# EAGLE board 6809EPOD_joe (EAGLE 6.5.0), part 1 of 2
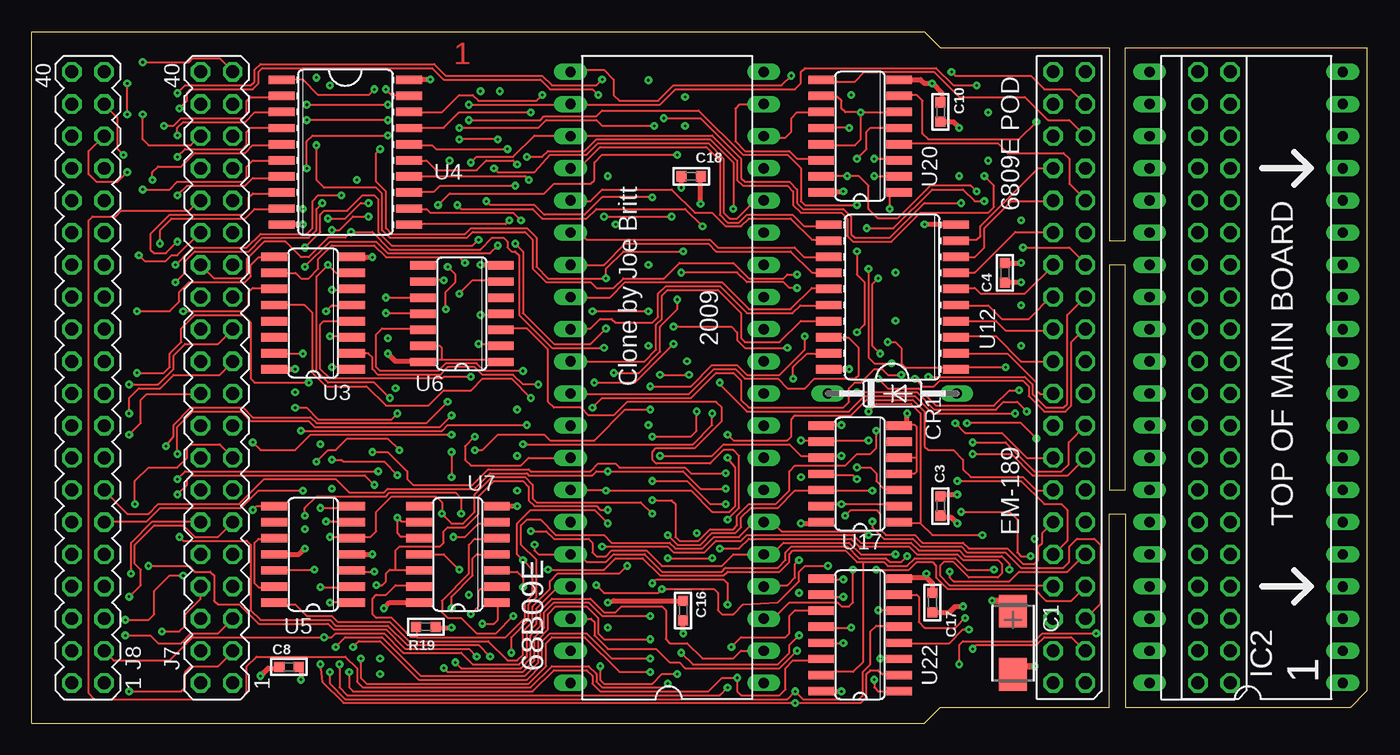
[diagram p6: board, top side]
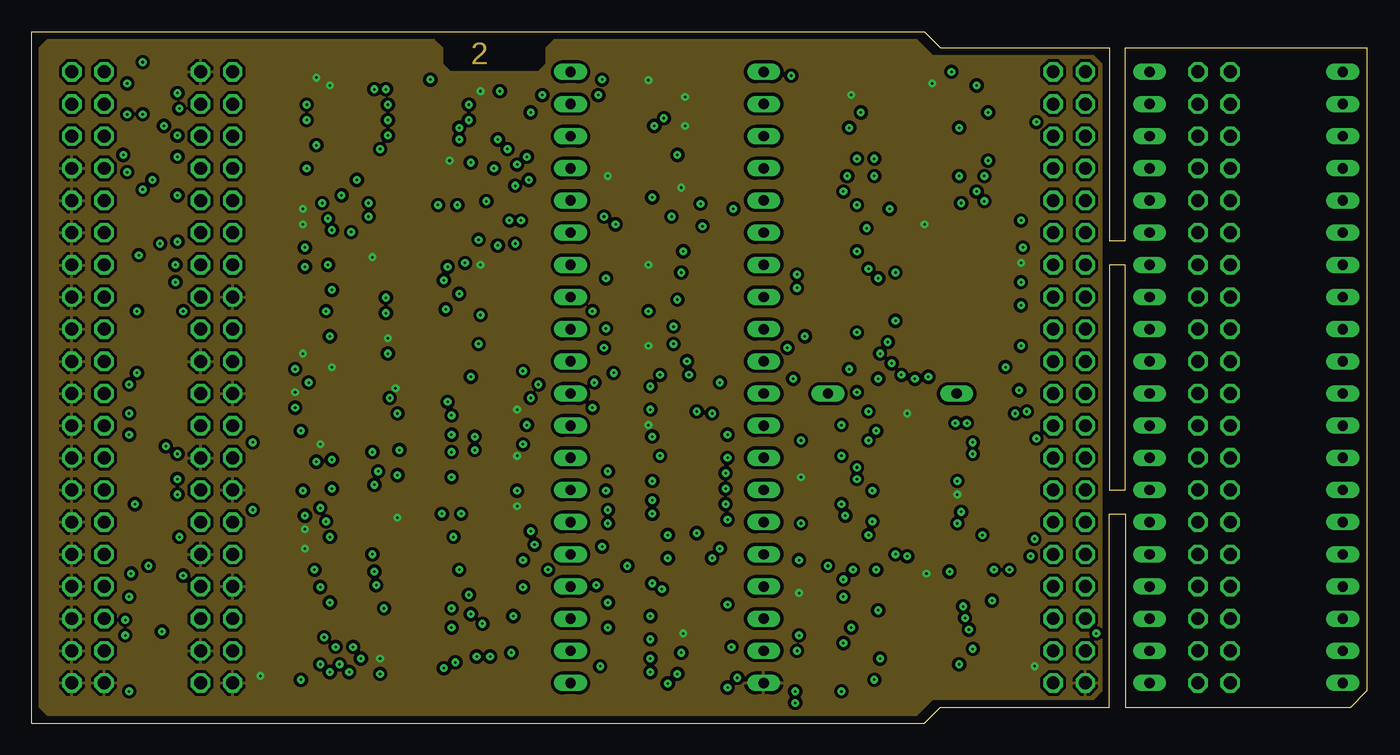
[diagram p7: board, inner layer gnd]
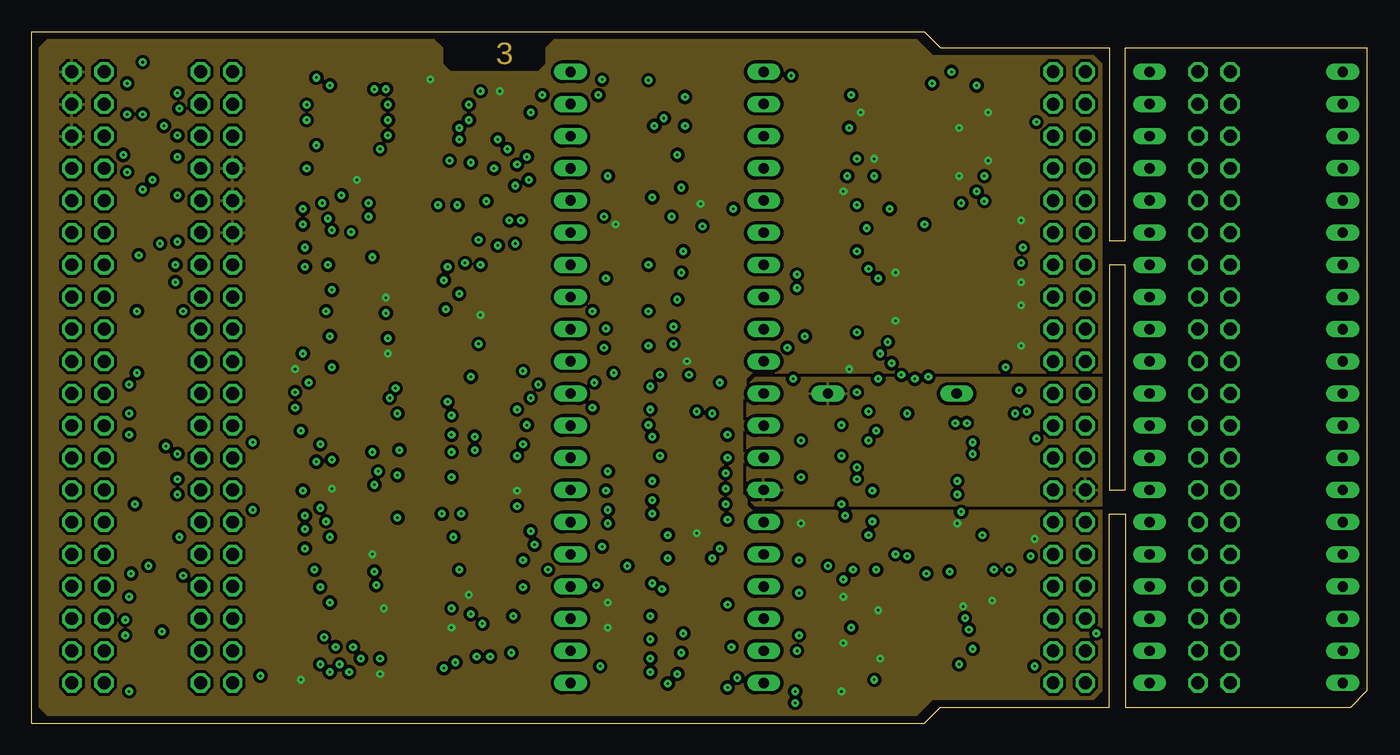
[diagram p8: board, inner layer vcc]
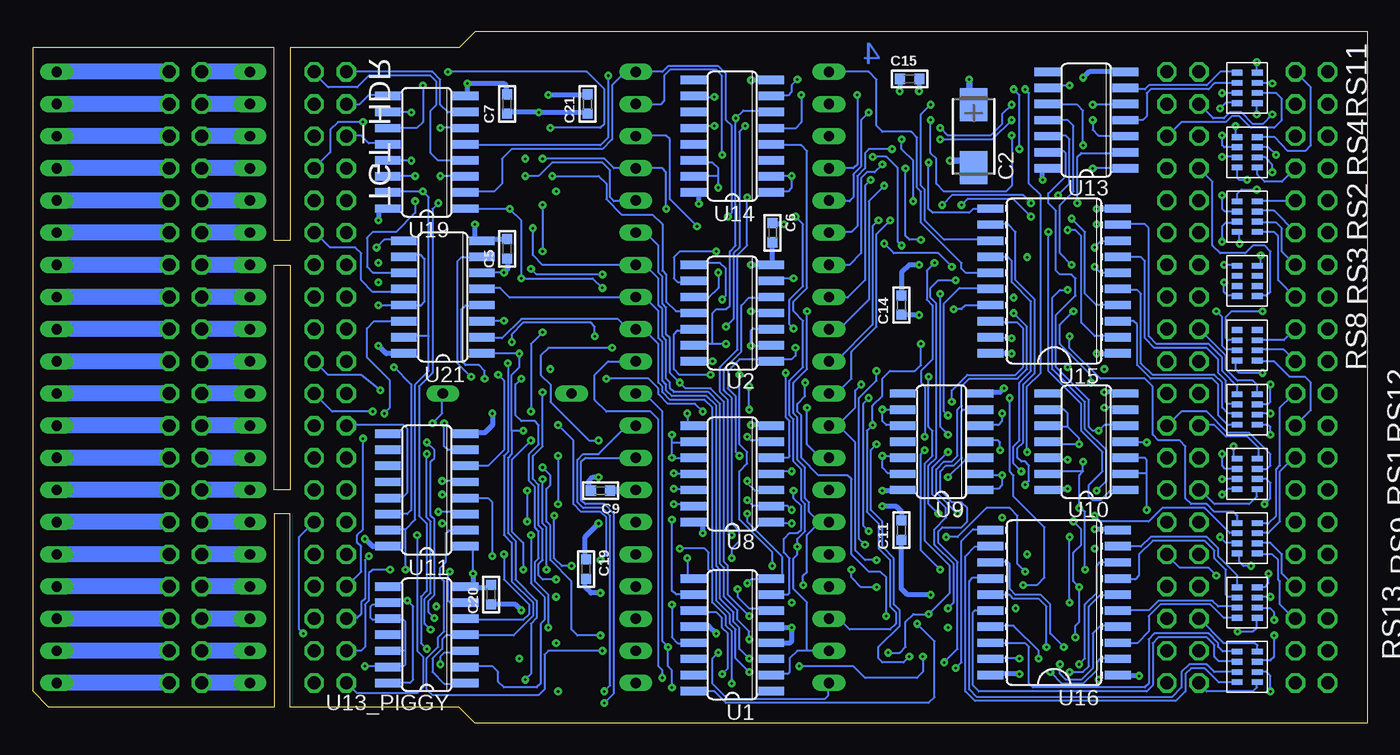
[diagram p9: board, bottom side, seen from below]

Size 105.41 x 54.61 mm. Coordinates in mm from the lower left corner, seen from the top.
Outline: 0,0 0,54.61 70.48,54.61 71.75,53.34 85.09,53.34 85.09,38.1 86.36,38.1 86.36,53.34 105.41,53.34 105.41,2.54 104.14,1.27 86.36,1.27 86.36,16.51 85.09,16.51 85.09,1.27 71.75,1.27 70.48,0 0,0
Outline: 85.09,18.41 86.36,18.41 86.36,36.2 85.09,36.2 85.09,18.41
Copper layers (1*4*5*16): Top 0.035mm / dielectric 1.5mm / gnd 0.035mm / dielectric 0.15mm / vcc 0.035mm / dielectric 0.2mm / Bottom 0.035mm
Design rules "default": minimum track width 6mil, minimum drill 8mil, track to track 6mil, track to pad 6mil, pad to pad 6mil, via to via 10mil, smd to smd 6mil, copper to edge 18mil, drill to drill 6mil, minimum pad ring 10mil, minimum via ring 8mil, stop-mask expansion 4mil, vias tented up to drill 8mil, thermal gap 10mil

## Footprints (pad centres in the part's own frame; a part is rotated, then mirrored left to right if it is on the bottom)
DIL40 = drill 0.813 long: 1 -24.13,-7.62; 2 -21.59,-7.62; 3 -19.05,-7.62; 4 -16.51,-7.62; 5 -13.97,-7.62; 6 -11.43,-7.62; 7 -8.89,-7.62; 8 -6.35,-7.62; 9 -3.81,-7.62; 10 -1.27,-7.62; 11 1.27,-7.62; 12 3.81,-7.62; 13 6.35,-7.62; 14 8.89,-7.62; 15 11.43,-7.62; 16 13.97,-7.62; 17 16.51,-7.62; 18 19.05,-7.62; 19 21.59,-7.62; 20 24.13,-7.62; 21 24.13,7.62; 22 21.59,7.62; 23 19.05,7.62; 24 16.51,7.62; 25 13.97,7.62; 26 11.43,7.62; 27 8.89,7.62; 28 6.35,7.62; 29 3.81,7.62; 30 1.27,7.62; 31 -1.27,7.62; 32 -3.81,7.62; 33 -6.35,7.62; 34 -8.89,7.62; 35 -11.43,7.62; 36 -13.97,7.62; 37 -16.51,7.62; 38 -19.05,7.62; 39 -21.59,7.62; 40 -24.13,7.62
CT6032 = smd 2.6 x 2.2: + 2.5,0; - -2.5,0
C0603 = smd 0.8 x 0.8: 1 -0.762,0; 2 0.762,0
DO35-10 = drill 0.813 long: A 5.08,0; C -5.08,0
HDR40 = drill 1.016 octagon: 1 -24.13,-1.27; 2 -21.59,-1.27; 3 -19.05,-1.27; 4 -16.51,-1.27; 5 -13.97,-1.27; 6 -11.43,-1.27; 7 -8.89,-1.27; 8 -6.35,-1.27; 9 -3.81,-1.27; 10 -1.27,-1.27; 11 1.27,-1.27; 12 3.81,-1.27; 13 6.35,-1.27; 14 8.89,-1.27; 15 11.43,-1.27; 16 13.97,-1.27; 17 16.51,-1.27; 18 19.05,-1.27; 19 21.59,-1.27; 20 24.13,-1.27; 21 24.13,1.27; 22 21.59,1.27; 23 19.05,1.27; 24 16.51,1.27; 25 13.97,1.27; 26 11.43,1.27; 27 8.89,1.27; 28 6.35,1.27; 29 3.81,1.27; 30 1.27,1.27; 31 -1.27,1.27; 32 -3.81,1.27; 33 -6.35,1.27; 34 -8.89,1.27; 35 -11.43,1.27; 36 -13.97,1.27; 37 -16.51,1.27; 38 -19.05,1.27; 39 -21.59,1.27; 40 -24.13,1.27
MA20-2 = drill 1.016 octagon: 1 -24.13,-1.27; 2 -24.13,1.27; 3 -21.59,-1.27; 4 -21.59,1.27; 5 -19.05,-1.27; 6 -19.05,1.27; 7 -16.51,-1.27; 8 -16.51,1.27; 9 -13.97,-1.27; 10 -13.97,1.27; 11 -11.43,-1.27; 12 -11.43,1.27; 13 -8.89,-1.27; 14 -8.89,1.27; 15 -6.35,-1.27; 16 -6.35,1.27; 17 -3.81,-1.27; 18 -3.81,1.27; 19 -1.27,-1.27; 20 -1.27,1.27; 21 1.27,-1.27; 22 1.27,1.27; 23 3.81,-1.27; 24 3.81,1.27; 25 6.35,-1.27; 26 6.35,1.27; 27 8.89,-1.27; 28 8.89,1.27; 29 11.43,-1.27; 30 11.43,1.27; 31 13.97,-1.27; 32 13.97,1.27; 33 16.51,-1.27; 34 16.51,1.27; 35 19.05,-1.27; 36 19.05,1.27; 37 21.59,-1.27; 38 21.59,1.27; 39 24.13,-1.27; 40 24.13,1.27
R0603 = smd 0.8 x 0.8: 1 -0.762,0; 2 0.762,0
V8V = smd 0.45 x 0.85: R1A -1.2,-0.8; R1B -1.2,0.8; R2A -0.4,-0.8; R2B -0.4,0.8; R3A 0.4,-0.8; R3B 0.4,0.8; R4A 1.2,-0.8; R4B 1.2,0.8
SO16 = smd 0.66 x 2.032: 1 -4.445,-3.073; 2 -3.175,-3.073; 3 -1.905,-3.073; 4 -0.635,-3.073; 5 0.635,-3.073; 6 1.905,-3.073; 7 3.175,-3.073; 8 4.445,-3.073; 9 4.445,3.073; 10 3.175,3.073; 11 1.905,3.073; 12 0.635,3.073; 13 -0.635,3.073; 14 -1.905,3.073; 15 -3.175,3.073; 16 -4.445,3.073
SO14 = smd 0.66 x 2.032: 1 -3.81,-3.073; 2 -2.54,-3.073; 3 -1.27,-3.073; 4 0,-3.073; 5 1.27,-3.073; 6 2.54,-3.073; 7 3.81,-3.073; 8 3.81,3.073; 9 2.54,3.073; 10 1.27,3.073; 11 0,3.073; 12 -1.27,3.073; 13 -2.54,3.073; 14 -3.81,3.073
SO20W = smd 0.66 x 2.032: 1 -5.715,-5.029; 2 -4.445,-5.029; 3 -3.175,-5.029; 4 -1.905,-5.029; 5 -0.635,-5.029; 6 0.635,-5.029; 7 1.905,-5.029; 8 3.175,-5.029; 9 4.445,-5.029; 10 5.715,-5.029; 11 5.715,5.029; 12 4.445,5.029; 13 3.175,5.029; 14 1.905,5.029; 15 0.635,5.029; 16 -0.635,5.029; 17 -1.905,5.029; 18 -3.175,5.029; 19 -4.445,5.029; 20 -5.715,5.029

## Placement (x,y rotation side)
68B09E  [DIL40]  50.16,27.3 90 top
C1  33uF  [CT6032]  77.47,6.35 90 top
C2  33uF  [CT6032]  31.12,46.35 90 bottom
C3  .1uF  [C0603]  71.75,17.14 90 top
C4  .1uF  [C0603]  76.83,35.56 90 top
C5  .1uF  [C0603]  67.94,37.46 90 bottom
C6  .1uF  [C0603]  46.99,38.73 270 bottom
C7  .1uF  [C0603]  67.94,48.89 90 bottom
C8  .1uF  [C0603]  20.32,4.44 180 top
C9  .1uF  [C0603]  60.58,18.36 180 bottom
C10  .1uF  [C0603]  71.75,48.26 90 top
C11  .1uF  [C0603]  36.83,15.24 90 bottom
C14  .1uF  [C0603]  36.83,33.02 90 bottom
C15  .1uF  [C0603]  36.17,50.88 0 bottom
C16  .1uF  [C0603]  51.44,8.89 270 top
C17  .1uF  [C0603]  71.12,9.53 90 top
C18  .1uF  [C0603]  52.07,43.18 180 top
C19  .1uF  [C0603]  61.72,12.17 270 bottom
C20  .1uF  [C0603]  69.22,10.16 90 bottom
C21  .1uF  [C0603]  61.59,48.89 90 bottom
CR1  1N4148  [DO35-10]  67.94,26.04 0 top
IC1  [DIL40]  95.89,27.3 90 top
IC2  [HDR40]  93.34,27.3 90 top
J7  [MA20-2]  14.61,27.3 90 top
J8  [MA20-2]  4.44,27.3 90 top
R19  10k  [R0603]  31.12,7.62 0 top
RS1  75  [V8V]  9.53,14.61 90 bottom
RS2  22  [V8V]  9.53,40 90 bottom
RS3  75  [V8V]  9.53,29.84 90 bottom
RS4  22  [V8V]  9.53,45.09 90 bottom
RS8  75  [V8V]  9.53,34.92 90 bottom
RS9  75  [V8V]  9.53,19.68 270 bottom
RS10  75  [V8V]  9.53,4.44 270 bottom
RS11  75  [V8V]  9.53,50.16 270 bottom
RS12  75  [V8V]  9.53,24.77 270 bottom
RS13  75  [V8V]  9.53,9.53 270 bottom
TGT_HDR  [HDR40]  81.91,27.3 90 top
U1  74LS75D  [SO16]  50.16,6.99 90 bottom
U2  74LS27D  [SO14]  50.16,32.38 90 bottom
U3  74LS367D  [SO16]  22.22,32.38 90 top
U4  74LS245DW  [SO20W]  24.77,45.09 270 top
U5  74LS73D  [SO14]  22.22,13.34 90 top
U6  74LS74D  [SO14]  33.96,32.33 90 top
U7  74LS32D  [SO14]  33.66,13.34 90 top
U8  74LS00D  [SO14]  50.16,19.68 90 bottom
U9  74LS00D  [SO14]  33.66,22.22 90 bottom
U10  74LS10D  [SO14]  22.22,22.22 90 bottom
U11  74LS367D  [SO16]  74.3,18.41 90 bottom
U12  74LS245DW  [SO20W]  67.94,33.66 90 top
U13  74LS04D  [SO14]  22.22,47.62 90 bottom
U13_PIGGY  74LS08D  [SO14]  74.3,6.99 90 bottom
U14  74LS367D  [SO16]  50.16,46.35 90 bottom
U15  74LS244DW  [SO20W]  24.77,34.92 90 bottom
U16  74LS244DW  [SO20W]  24.77,9.53 90 bottom
U17  74LS32D  [SO14]  65.41,19.68 90 top
U19  74LS257D  [SO16]  74.3,45.09 90 bottom
U20  74LS257D  [SO16]  65.41,46.35 90 top
U21  74LS257D  [SO16]  73.03,33.66 90 bottom
U22  74LS257D  [SO16]  65.41,6.99 90 top

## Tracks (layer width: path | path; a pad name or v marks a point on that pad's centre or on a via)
A0  (via drill 0.2)
  Top 0.152: v22.78,4.65 22.94,3.28 24.61,1.6 v60.27,1.6 65.46,1.6 65.91,2.06 65.91,3.89 66.22,4.19 66.83,4.19 67.13,3.89 68.4,3.89 U22.2
  Bottom 0.152: U16.8 19.76,12.73 21.11,12.73 21.41,12.42 21.41,10.29 22.33,9.37 22.33,5.1 v22.78,4.65 | v60.27,1.6 59.51,2.36 59.51,16.54 60.27,17.3 61.8,17.3 62.1,17.6 62.1,20.65 61.8,20.95 68B09E.8
A1  (via drill 0.2)
  Top 0.152: v23.55,4.04 23.55,3.12 24.77,1.91 59.66,1.91 v60.27,2.51 60.88,1.91 65.3,1.91 65.61,2.21 65.61,4.04 66.22,4.65 66.22,7.24 66.67,7.7 68.5,7.7 68.5,7.65 U22.5
  Bottom 0.152: U16.6 19.76,10.13 21.11,10.13 22.02,9.22 22.02,4.5 22.48,4.04 v23.55,4.04 | v60.27,2.51 59.82,2.97 59.82,16.38 60.43,16.99 61.95,16.99 62.41,17.45 62.41,20.8 61.95,21.26 60.73,21.26 58.45,23.55 57.84,23.55 68B09E.9
A2  (via drill 0.2)
  Top 0.152: v24.31,4.65 24.31,2.82 24.92,2.21 54.33,2.21 v54.94,2.82 | v55.24,6.02 56.01,6.78 59.51,6.78 59.82,7.09 59.82,8.46 60.27,8.92 62.25,8.92 62.28,8.89 U22.11
  Bottom 0.152: U16.4 19.81,7.7 21.11,7.7 21.72,7.09 21.72,4.34 22.63,3.43 23.85,3.43 24.31,3.89 v24.31,4.65 | v54.94,2.82 54.94,4.19 55.24,4.5 v55.24,6.02 55.7,6.48 55.7,24.61 57.07,25.98 57.68,25.98 68B09E.10
A3  (via drill 0.2)
  Top 0.152: v25.07,4.04 25.07,2.82 25.38,2.51 39.55,2.51 41.22,4.19 43.81,4.19 44.27,3.73 44.27,3.12 44.88,2.51 53.42,2.51 54.48,3.58 v55.7,3.58 55.7,2.51 56.01,2.21 59.05,2.21 59.51,2.67 59.51,4.34 60.12,4.95 62.15,4.95 U22.14
  Bottom 0.152: U16.2 19.76,5.1 21.11,5.1 21.41,4.8 21.41,4.19 22.48,3.12 24.15,3.12 v25.07,4.04 | v55.7,3.58 55.7,4.19 56.01,4.5 56.01,24 56.62,24.61 60.12,24.61 61.04,25.53 61.04,27.51 59.97,28.57 68B09E.11
A4  (via drill 0.2)
  Top 0.152: v48.84,4.04 46.41,4.04 43.66,6.78 41.07,6.78 40.62,6.33 40.62,4.5 39.24,3.12 26.44,3.12 25.98,3.58 v25.98,5.1
  Bottom 0.152: U16.17 29.87,7.7 27.96,7.7 25.98,5.71 v25.98,5.1 | U21.2 69.88,30.4 68.35,30.4 66.83,31.93 59.21,31.93 58.45,31.17 57.84,31.17 68B09E.12 57.73,31.12 57.68,31.17 57.07,31.01 56.01,29.95 56.01,26.9 55.7,26.59 55.7,26.14 55.09,25.53 52.35,25.53 51.74,24.92 51.74,12.27 51.44,11.96 51.44,9.68 50.37,8.61 50.37,7.85 49.91,7.39 49.91,5.1 v48.84,4.04
A5  (via drill 0.2)
  Top 0.152: v48.84,5.1 45.8,5.1 43.81,7.09 40.92,7.09 40.31,6.48 40.31,4.65 39.09,3.43 30.56,3.43 27.51,6.48 25.83,6.48 v25.38,6.02
  Bottom 0.152: U16.15 29.82,10.13 28.27,10.13 27.96,9.83 25.98,9.83 25.38,9.22 v25.38,6.02 | U21.5 69.88,34.37 68.5,34.37 67.74,33.6 57.89,33.6 68B09E.13 57.73,33.66 57.68,33.6 57.07,33.6 56.01,32.54 56.01,30.4 55.7,30.1 55.7,27.05 55.4,26.75 55.4,26.29 54.94,25.83 52.2,25.83 51.44,25.07 51.44,12.42 51.13,12.12 51.13,9.83 50.06,8.76 50.06,8 49.61,7.54 49.61,5.87 v48.84,5.1
A6  (via drill 0.2)
  Top 0.152: v75.21,41.22 74.45,41.22 73.53,42.14 71.09,42.14 68.05,39.09 v65.91,39.09 | v48.84,6.63 45.19,6.63 44.73,7.09 44.73,8.31 43.81,9.22 41.38,9.22 40.77,8.61 40.77,7.39 40,6.63 40,4.8 38.94,3.73 30.71,3.73 27.66,6.78 24.77,6.78 v24,6.02
  Bottom 0.152: U16.13 29.82,12.73 28.42,12.73 28.27,12.57 28.27,10.59 27.81,10.13 25.83,10.13 25.07,9.37 25.07,7.09 v24,6.02 | U21.11 76.12,35.59 78.56,35.59 79.02,36.04 79.02,38.33 78.56,38.79 76.73,38.79 75.21,40.31 v75.21,41.22 | v65.91,39.09 65.91,36.96 65.15,36.2 68B09E.14 57.07,36.2 56.01,35.13 56.01,32.99 55.7,32.69 55.7,30.56 55.4,30.25 55.4,27.2 55.09,26.9 55.09,26.44 54.79,26.14 52.05,26.14 51.13,25.22 51.13,12.57 50.82,12.27 50.82,9.98 49.76,8.92 49.76,8.15 48.84,7.24 v48.84,6.63
A7  (via drill 0.2)
  Top 0.152: v77.65,24.46 71.09,24.46 69.72,25.83 65.76,25.83 64.54,24.61 56.46,24.61 54.33,26.75 v54.33,26.9 | v48.84,8.46 45.03,8.46 43.97,9.53 41.22,9.53 40.46,8.76 40.46,7.54 39.7,6.78 39.7,4.95 38.79,4.04 32.84,4.04 v32.54,4.34
  Bottom 0.152: U16.11 29.87,15.32 31.17,15.32 32.08,14.4 32.08,4.8 v32.54,4.34 | 68B09E.15 57.84,38.79 57.07,38.79 56.01,37.72 56.01,35.59 55.7,35.28 55.7,33.15 55.4,32.84 55.4,30.71 55.09,30.4 55.09,27.66 v54.33,26.9 53.87,26.44 51.89,26.44 50.82,25.38 50.82,12.73 50.52,12.42 50.52,10.13 v48.84,8.46 | U21.14 78.44,31.75 79.02,31.17 79.02,28.88 77.19,27.05 77.19,24.92 v77.65,24.46
A8  (via drill 0.2)
  Top 0.152: U20.2 68.45,43.2 v66.52,43.2 | v21.56,37.57 22.78,38.79 22.78,40.16 23.09,40.46 24.92,40.46 26.14,41.68 27.05,41.68 27.36,41.38 27.36,38.79 28.42,37.72 34.82,37.72 v35.28,38.18 | v36.5,43.81 36.8,43.51 39.7,43.51 40.92,44.88 43.81,44.88 44.73,45.8 53.42,45.8 54.63,44.58 54.63,40.31 55.09,39.85 55.7,39.85 57.07,41.22 57.68,41.22 57.73,41.27 68B09E.16
  Bottom 0.152: 68B09E.16 57.84,41.22 59.51,41.22 59.82,41.53 59.82,43.66 60.43,44.27 64.39,44.27 65.46,43.2 v66.52,43.2 | U15.8 19.81,38.02 21.11,38.02 v21.56,37.57 | v35.28,38.18 36.2,38.18 36.5,38.48 v36.5,43.81
A9  (via drill 0.2)
  Top 0.152: U20.5 68.45,47.02 66.22,47.02 65.91,46.71 65.91,45.34 v65.15,44.58 | v21.56,36.04 23.55,38.02 27.2,38.02 28.12,37.11 36.2,37.11 v36.8,37.72 | v39.09,44.73 40.31,44.73 40.77,45.19 43.66,45.19 44.58,46.1 53.57,46.1 55.4,44.27 v55.4,40.62
  Bottom 0.152: v65.15,44.58 60.27,44.58 59.51,43.81 68B09E.17 55.7,43.81 55.4,43.51 v55.4,40.62 | U15.6 21.08,35.56 v21.56,36.04 | v36.8,37.72 37.11,38.02 37.11,43.81 38.02,44.73 v39.09,44.73
A10  (via drill 0.2)
  Top 0.152: 68B09E.18 57.89,46.25 59.51,46.25 59.97,46.71 59.97,47.78 60.43,48.23 62.31,48.23 U20.11 | v23.39,39.85 24.77,39.85 25.98,41.07 v26.59,41.07 | v33.6,40.92 33.91,40.62 39.55,40.62 40.31,39.85 43.81,39.85 44.58,40.62 51.59,40.62 v52.96,39.24
  Bottom 0.152: U15.4 21.44,33.02 22.33,33.91 22.33,38.79 v23.39,39.85 | v26.59,41.07 27.2,41.68 32.84,41.68 v33.6,40.92 | v52.96,39.24 55.09,41.38 55.09,46.1 55.4,46.41 57.68,46.41 57.73,46.35 68B09E.18
A11  (via drill 0.2)
  Top 0.152: U20.14 62.2,44.58 60.43,44.58 59.82,45.19 56.31,45.19 55.55,45.95 55.55,48.54 55.85,48.84 57.73,48.84 68B09E.19 | v23.7,38.94 24.31,38.94 25.38,40 v26.59,40 | v32.08,40.92 32.99,41.83 40.46,41.83 41.22,42.6 44.12,42.6 44.42,42.9 44.42,44.27 45.03,44.88 v50.98,44.88
  Bottom 0.152: U15.2 20.27,30.48 20.5,30.56 21.56,30.56 22.63,31.62 22.63,38.48 23.09,38.94 v23.7,38.94 | v26.59,40 27.96,41.38 31.62,41.38 v32.08,40.92 | v50.98,44.88 50.98,51.13 51.44,51.59 55.09,51.59 55.55,51.13 55.55,49.15 55.85,48.84 57.84,48.84 68B09E.19
A12  (via drill 0.2)
  Top 0.152: v32.69,32.69 32.69,34.06 33.45,34.82 33.45,35.43 v32.84,36.04 | v45.34,31.17 44.12,29.95 41.22,29.95 38.79,32.38 38.79,37.26 v38.18,37.87 | v45.19,40 v50.52,40
  Bottom 0.152: U19.2 71.14,41.99 68.96,41.99 68.35,42.6 68.35,44.58 67.59,45.34 60.43,45.34 59.66,46.1 59.66,50.37 58.6,51.44 68B09E.20 55.7,51.44 55.24,51.89 51.28,51.89 50.67,51.28 50.67,47.62 50.22,47.17 50.22,40.31 v50.52,40 | U15.17 29.82,32.99 31.77,32.99 32.08,32.69 v32.69,32.69 | v45.34,31.17 45.64,31.47 45.64,33.45 44.58,34.52 44.58,39.39 v45.19,40 | v38.18,37.87 37.41,37.11 33.91,37.11 v32.84,36.04
A13  (via drill 0.2)
  Top 0.152: 68B09E.21 42.7,51.59 45.19,51.59 45.95,50.82 45.95,49.61 46.41,49.15 49.45,49.15 50.67,50.37 59.21,50.37 v59.97,51.13
  Bottom 0.152: v59.97,51.13 59.97,46.25 60.58,45.64 71.14,45.64 U19.5 | U15.15 31.75,35.56 32.08,35.89 32.08,36.35 35.28,39.55 35.28,41.99 35.59,42.29 35.59,46.25 36.04,46.71 38.33,46.71 38.79,47.17 38.79,50.82 39.39,51.44 68B09E.21
A14  (via drill 0.2)
  Top 0.152: v74.6,50.37 72.77,50.37 71.4,51.74 61.04,51.74 60.73,51.44 60.73,50.52 60.27,50.06 50.82,50.06 49.61,48.84 42.49,48.84 | 42.49,48.84 68B09E.22 | v34.52,48.84 42.49,48.84
  Bottom 0.152: U19.11 75.08,46.99 74.6,47.47 v74.6,50.37 | U15.13 29.87,38.18 33.45,38.18 34.98,39.7 34.98,42.14 35.28,42.44 35.28,48.08 v34.52,48.84
A15  (via drill 0.2)
  Top 0.152: v75.21,43.2 75.97,42.44 75.97,40.77 75.51,40.31 70.18,40.31 67.89,38.02 64.85,38.02 64.39,38.48 64.39,39.85 63.93,40.31 60.73,40.31 60.12,40.92 60.12,41.99 59.66,42.44 56.16,42.44 55.7,42.9 55.7,44.42 53.72,46.41 42.6,46.41 68B09E.23 42.49,46.41 39.7,46.41 38.02,44.73 35.13,44.73 v34.67,44.27
  Bottom 0.152: U19.14 77.34,43.2 v75.21,43.2 | U15.11 29.82,40.62 31.17,40.62 31.47,40.31 34.37,40.31 34.67,40.62 v34.67,44.27
AVMA'  (via drill 0.2)
  Top 0.152: U6.9 30.84,34.98 v32.54,34.98 | v21.56,16.38 21.56,16.99 22.48,17.91 27.96,17.91 28.27,18.21 33.45,18.21 33.91,17.75 v33.91,16.54
  Bottom 0.152: RS1.R3B 10.9,15.01 12.88,16.99 16.23,16.99 17.3,15.93 21.11,15.93 v21.56,16.38 | v33.91,16.54 34.67,17.3 34.67,20.34 34.06,20.95 34.06,33.15 34.52,33.6 34.52,34.37 33.91,34.98 v32.54,34.98
CPU_AVMA  (via drill 0.2)
  Top 0.152: U6.12 30.78,31.17 27.66,31.17 27.2,30.71 27.2,28.12 27.51,27.81 32.08,27.81 32.69,28.42 35.13,28.42 35.74,27.81 v38.79,27.81 | 42.6,13.34 43.2,13.34 43.81,12.73 45.34,12.73 45.95,13.34 48.39,13.34 49.76,11.96 54.48,11.96 54.79,12.27 58.9,12.27 59.51,12.88 59.51,13.49 59.97,13.95 64.39,13.95 65.3,13.03 67.44,13.03 67.74,12.73 68.66,12.73 v69.11,13.18 | v39.7,14.1 39.7,13.64 40,13.34 42.6,13.34 | 42.6,13.34 68B09E.36
  Bottom 0.152: v38.79,27.81 38.79,27.05 40.16,25.68 40.16,14.55 v39.7,14.1 | v69.11,13.18 69.11,17.45 69.42,17.75 70.94,17.75 70.97,17.78 U11.4
CPU_BA  (via drill 0.2)
  Top 0.152: v66.06,14.86 65.76,15.16 59.21,15.16 58.45,15.93 58.19,15.88 68B09E.6 57.02,15.88 55.85,14.71 53.87,14.71 52.96,13.79 50.82,13.79 50.37,14.25 45.8,14.25 45.19,14.86 41.38,14.86 40.16,16.08 39.09,16.08 38.63,15.62 38.63,14.1 39.85,12.88 39.85,9.98 39.24,9.37 39.24,8.15 37.87,6.78 v37.87,5.56 | U7.2 36.85,10.64 36.65,10.59 35.43,10.59 35.28,10.44 35.28,9.22 v34.67,8.61 | U3.4 23.06,31.75 22.78,31.47 22.78,27.96 23.55,27.2 32.38,27.2 32.54,27.36 v34.67,27.36
  Bottom 0.152: v66.06,14.86 66.06,11.05 65,9.98 65,8.15 65.3,7.85 65.3,3.12 65.61,2.82 68.2,2.82 68.66,3.28 68.66,4.04 69.11,4.5 70.94,4.5 70.99,4.44 U13_PIGGY.2 | v37.87,5.56 36.96,5.56 36.5,6.02 36.5,8 35.89,8.61 v34.67,8.61 32.99,10.29 32.99,12.42 34.98,14.4 34.98,20.5 34.37,21.11 34.37,23.09 34.67,23.39 v34.67,27.36
CPU_BA'  (via drill 0.2)
  Top 0.152: v8.31,27.66 10.44,27.66 10.9,28.12 10.9,29.18 11.81,30.1 11.81,31.17 12.88,32.23 16.69,32.23 17.3,31.62 17.3,27.2 17.6,26.9 v21.87,26.9 | U3.5 25.27,32.99 23.7,32.99 v23.24,32.54
  Bottom 0.152: RS3.R1B 10.37,28.64 10.44,28.57 10.44,27.96 10.13,27.66 v8.31,27.66 | v21.87,26.9 21.87,27.51 24.31,29.95 24.31,31.47 v23.24,32.54
CPU_BS  (via drill 0.2)
  Top 0.152: v68.2,13.34 65.46,13.34 64.54,14.25 59.36,14.25 58.45,13.34 68B09E.5 55.4,13.34 54.48,12.42 49.76,12.42 48.54,13.64 45.8,13.64 45.34,13.18 44.58,13.18 44.27,13.49 44.27,14.25 43.97,14.55 41.22,14.55 40.62,15.16 v39.39,15.16 | U3.12 21.54,33.02 22.17,32.38 22.17,27.66 23.24,26.59 26.44,26.59 27.96,25.07 31.32,25.07 32.54,26.29 34.67,26.29 35.59,27.2 37.87,27.2 v39.39,25.68
  Bottom 0.152: v68.2,13.34 68.2,11.35 66.22,9.37 66.22,8.61 66.67,8.15 71.25,8.15 71.22,8.28 U13_PIGGY.5 | v39.39,25.68 39.85,25.22 39.85,15.62 v39.39,15.16
CPU_BS'  (via drill 0.2)
  Top 0.152: v11.96,32.54 16.69,32.54 17.14,32.99 17.14,34.06 17.45,34.37 19.07,34.37 U3.11
  Bottom 0.152: v11.96,32.54 11.51,32.08 11.51,29.79 11.2,29.49 10.59,29.49 10.55,29.45 RS3.R2B
CPU_BUSY  (via drill 0.2)
  Top 0.152: v68.66,27.51 67.59,27.51 67.13,27.96 66.52,27.96 65.46,26.9 65,26.9 64.54,26.44 64.54,25.38 64.08,24.92 56.62,24.92 56.01,25.53 56.01,27.05 55.4,27.66 54.03,27.66 52.05,25.68 45.03,25.68 v44.27,24.92 | U3.10 20.83,35.56 21.26,35.13 21.87,35.13 22.63,35.89 22.63,36.65 23.7,37.72 27.05,37.72 27.96,36.8 33.76,36.8 v34.21,36.35 | 68B09E.33 39.24,20.95 38.63,20.34 34.67,20.34 34.21,20.8 34.21,21.87 v34.98,22.63
  Bottom 0.152: U11.6 69.44,20.32 68.2,21.56 68.2,27.05 v68.66,27.51 | v44.27,24.92 44.27,22.02 43.2,20.95 68B09E.33 | v34.21,36.35 34.82,35.74 34.82,33.45 34.37,32.99 34.37,28.73 35.28,27.81 35.28,26.9 34.98,26.59 v34.98,22.63
CPU_BUSY'  (via drill 0.2)
  Top 0.152: v8.31,32.54 10.9,32.54 11.66,33.3 11.66,34.06 12.42,34.82 16.84,34.82 17.3,35.28 17.3,36.2 17.91,36.8 19.13,36.8 U3.9
  Bottom 0.152: v8.31,32.54 10.74,32.54 11.2,32.08 11.2,30.4 11.05,30.25 10.44,30.25 10.43,30.24 RS3.R3B
CPU_E  (via drill 0.2)
  Top 0.152: 68B09E.34 42.6,18.36 v45.34,18.36 52.05,18.36 53.72,16.69 55.09,16.69 55.55,17.14 55.55,20.19 v54.94,20.95 | v54.94,22.78 55.4,22.33 59.66,22.33 59.97,22.63 59.97,24 60.27,24.31 64.69,24.31 65.91,25.53 69.57,25.53 70.48,24.61 70.48,21.87 70.79,21.56 72.77,21.56 73.53,20.8 73.53,20.04 74.14,19.43 78.26,19.43 79.32,18.36 80.54,18.36 80.59,18.41 TGT_HDR.34
  Bottom 0.152: v45.34,18.36 45.34,17.75 44.73,17.14 44.73,15.32 45.03,15.01 45.64,15.01 46.1,14.55 46.1,13.49 45.64,13.03 45.64,10.29 45.8,10.13 47.12,10.13 U1.7 | 53.11,20.95 U8.10 v54.94,20.95 54.94,22.17 | U8.9 53.16,22.22 53.11,22.17 54.94,22.17 | 54.94,22.17 v54.94,22.78
CPU_E'  (via drill 0.2)
  Top 0.152: v50.22,13.03 v53.72,13.03
  Bottom 0.152: U1.9 53.72,11.43 v53.72,13.03 | v50.22,13.03 50.22,13.79 49.61,14.4 49.61,15.16 50.22,15.77 50.22,25.68 50.82,26.29 50.82,27.96 49.45,29.34 49.45,32.99 48.84,33.6 47.14,33.6 U2.5
CPU_E*  (via drill 0.2)
  Top 0.152: v11.66,14.71 11.96,14.4 16.99,14.4 17.3,14.1 17.3,8.92 18.06,8.15 23.55,8.15 24,7.7 28.12,7.7 29.64,6.17 35.28,6.17 v36.2,5.26 | v38.79,22.02 52.2,22.02 53.72,23.55 v53.72,24.46
  Bottom 0.152: RS1.R2B 10.59,14.25 11.2,14.25 v11.66,14.71 | v36.2,5.26 36.65,4.8 38.33,4.8 38.63,5.1 38.63,6.02 36.96,7.7 36.96,8.92 37.41,9.37 37.41,13.03 38.33,13.95 38.33,15.93 39.24,16.84 39.24,21.56 v38.79,22.02 | U8.8 53.24,23.52 53.72,23.55 v53.72,24.46
CPU_E*'  (via drill 0.2)
  Top 0.152: v49,11.05 49.3,11.35 54.63,11.35 54.94,11.05 v54.94,9.37 | 25.2,14.71 U5.5 | v23.55,14.71 25.2,14.71 | U5.1 v23.55,9.53 | 25.2,14.71 26.75,14.71 27.2,15.16 27.2,16.69 28.42,17.91 31.93,17.91 32.38,17.45 v32.38,16.54 33.15,15.77 34.06,15.77 34.98,16.69 34.98,18.06 36.35,19.43 38.94,19.43 39.55,18.82 39.55,17.75 39.85,17.45 48.08,17.45 v49,16.54 | U6.11 31.12,32.33 31.17,32.38 v27.96,32.38
  Bottom 0.152: 46.25,11.2 U1.8 | v54.94,9.37 54.94,6.78 54.48,6.33 53.26,6.33 U1.13 | v23.55,9.53 v23.55,14.71 | v32.38,16.54 34.06,18.21 34.06,20.04 33.45,20.65 32.84,20.65 32.38,21.11 32.38,24.77 32.08,25.07 32.08,26.59 31.47,27.2 27.66,27.2 26.9,27.96 26.9,31.32 v27.96,32.38 | 46.25,11.2 46.86,11.2 47.02,11.35 48.69,11.35 v49,11.05 | v49,16.54 49,15.93 46.25,13.18 46.25,11.2
CPU_FIRQ*  (via drill 0.2)
  Top 0.152: 68B09E.4 57.89,10.9 59.66,10.9 60.27,11.51 60.27,12.57 v60.58,12.88 | U17.8 62.38,23.55 v63.93,23.55
  Bottom 0.152: v60.58,12.88 60.12,13.34 60.12,16.23 60.58,16.69 62.1,16.69 62.71,17.3 62.71,22.33 v63.93,23.55
CPU_HALT*  (via drill 0.2)
  Top 0.152: v51.28,5.56 52.2,4.65 58.9,4.65 59.82,5.56 59.82,6.17 v60.58,6.93 | v65.15,20.19 66.22,20.19 66.67,19.74 66.67,19.13 67.28,18.52 68.38,18.52 U17.3
  Bottom 0.152: 68B09E.40 42.6,3.12 42.6,2.21 42.9,1.91 50.52,1.91 51.74,3.12 51.74,5.1 v51.28,5.56 | v60.58,6.93 62.41,6.93 62.86,7.39 62.86,11.2 64.54,12.88 64.54,15.62 64.85,15.93 64.85,18.52 64.54,18.82 64.54,19.58 v65.15,20.19
CPU_IRQ*  (via drill 0.2)
  Top 0.152: 68B09E.3 57.84,8.31 58.6,8.31 59.82,9.53 63.63,9.53 63.93,9.22 64.54,9.22 64.85,9.53 v64.85,12.12 | U17.11 62.53,19.58 64.85,19.58 v65.15,19.28
  Bottom 0.152: v64.85,12.12 64.85,15.47 65.15,15.77 v65.15,19.28
CPU_LIC  (via drill 0.2)
  Top 0.152: 68B09E.38 44.17,8.26 44.42,8 44.42,6.93 45.49,5.87 49.3,5.87 50.37,4.8 51.13,4.8 51.59,4.34 59.05,4.34 v60.43,5.71 | v21.26,23.09 32.38,23.09 32.84,23.55 v39.09,23.55 | U6.2 37.19,29.95 v35.28,29.95
  Bottom 0.152: U11.2 72.54,15.24 72.77,15.01 72.77,12.73 73.23,12.27 73.23,11.51 72.92,11.2 72.92,7.24 73.38,6.78 73.38,6.02 74.3,5.1 74.3,2.67 73.84,2.21 65.46,2.21 65,2.67 65,5.41 64.69,5.71 v60.43,5.71 | U13.13 25.2,45.19 24,45.19 23.85,45.03 23.85,43.2 25.22,41.83 25.22,41.07 24.61,40.46 24.61,35.74 24.31,35.43 23.39,35.43 23.09,35.13 23.09,33.76 24.61,32.23 24.61,28.12 22.02,25.53 22.02,23.39 21.72,23.09 v21.26,23.09 20.8,23.55 19.74,23.55 19.63,23.49 U10.5 | 68B09E.38 41.88,8.26 41.68,8.15 40.92,7.39 37.72,7.39 37.26,7.85 37.26,8.76 37.72,9.22 37.72,12.88 38.63,13.79 38.63,15.77 39.55,16.69 39.55,23.09 v39.09,23.55 39.09,25.07 38.33,25.83 38.33,27.2 37.72,27.81 35.74,27.81 35.28,28.27 v35.28,29.95
CPU_NMI*  (via drill 0.2)
  Top 0.152: v33.45,4.8 33.91,4.34 38.63,4.34 39.39,5.1 39.39,6.93 40.16,7.7 40.16,8.92 41.07,9.83 44.12,9.83 45.19,8.76 46.1,8.76 46.56,9.22 49.76,9.22 50.06,8.92 50.06,6.63 50.37,6.33 51.74,6.33 52.96,5.1 55.4,5.1 56.01,5.71 68B09E.2
  Bottom 0.152: v33.45,4.8 32.38,5.87 32.38,12.73 33.91,14.25 33.91,15.16 33.6,15.47 32.08,15.47 31.62,15.93 31.62,16.99 32.08,17.45 32.84,17.45 33.76,18.36 33.76,19.89 33.3,20.34 32.69,20.34 32.08,20.95 32.08,24.61 31.93,24.77 U9.6
CPU_Q  (via drill 0.2)
  Top 0.152: v62.86,12.42 61.04,12.42 60.58,11.96 60.58,11.2 58.9,9.53 56.16,9.37 55.4,8.61 54.48,8.61 54.18,8.92 54.18,10.29 53.87,10.59 v49.76,10.59 49.45,10.29 45.19,10.29 v44.58,10.9 | v44.27,32.54 v48.69,32.54 | TGT_HDR.35 79.78,15.01 79.78,14.25 79.48,13.95 79.48,12.88 79.17,12.57 78.26,12.57 77.04,13.79 73.99,13.79 73.53,14.25 70.33,14.25 69.72,14.86 67.44,14.86 66.98,15.32 66.98,16.54 66.67,16.84 64.69,16.84 v64.24,16.38
  Bottom 0.152: U1.6 47.12,9.07 48.84,9.07 49.76,9.98 v49.76,10.59 | v62.86,12.42 63.63,12.42 64.24,13.03 v64.24,16.38 | v44.58,10.9 44.58,11.66 44.27,11.96 44.27,14.86 43.26,15.88 68B09E.35 43.31,15.88 44.12,16.69 44.12,17.45 44.42,17.75 44.42,20.19 45.03,20.8 45.03,24.15 45.34,24.46 45.34,26.9 44.27,27.96 v44.27,32.54 | v48.69,32.54 47.24,32.54 U2.4
CPU_Q'  (via drill 0.2)
  Top 0.152: U6.3 36.78,31.17 39.09,31.17 40.77,29.49 40.77,25.38 41.22,24.92 43.36,24.92 43.97,24.31 45.95,24.31 47.02,25.38 54.03,25.38 54.48,24.92 54.48,23.85 52.35,21.72 49.3,21.72 49,21.41 49,20.8 49.3,20.5 53.57,20.5 54.63,21.56 55.4,21.56 55.85,21.11 55.85,16.99 v54.94,16.08
  Bottom 0.152: U1.10 54.61,10.16 54.94,10.44 v54.94,16.08
CPU_Q*'  (via drill 0.2)
  Top 0.152: v9.22,12.42 12.42,12.42 12.88,11.96 14.1,11.96 14.4,11.66 14.4,9.68 14.71,9.37 16.38,9.37 17.91,7.85 23.39,7.85 23.85,7.39 27.96,7.39 29.49,5.87 34.52,5.87 v35.13,5.26 | v44.88,4.5 44.88,3.43 45.19,3.12 49,3.12 49.76,3.89 v50.98,3.89
  Bottom 0.152: RS1.R1B 10.13,13.41 10.13,12.73 9.83,12.42 v9.22,12.42 | v35.13,5.26 35.13,4.04 35.59,3.58 39.7,3.58 40.62,4.5 v44.88,4.5 | U1.11 53.11,8.76 51.44,8.76 50.98,8.31 50.98,7.54 50.52,7.09 50.52,4.34 v50.98,3.89
CPU_R/W  (via drill 0.2)
  Top 0.152: U3.2 26.57,29.21 26.9,28.88 26.9,27.96 27.36,27.51 32.23,27.51 32.84,28.12 34.98,28.12 35.59,27.51 38.02,27.51 38.79,26.75 v40,26.75 | 30.4,6.78 29.95,6.78 28.42,8.31 27.2,8.31 26.9,8.61 26.9,9.83 27.2,10.13 27.96,10.13 28.73,10.9 30.68,10.9 U7.13 | 30.4,6.78 37.41,6.78 38.94,8.31 38.94,9.53 39.55,10.13 39.55,12.12 v38.79,12.88 38.33,13.34 38.33,15.77 39.39,16.84 44.42,16.84 v45.49,15.77 | R19.1 30.4,7.57 30.4,6.78
  Bottom 0.152: v40,26.75 40.46,26.29 40.46,24.92 41.83,23.55 | 68B09E.32 42.49,23.49 42.44,23.55 41.83,23.55 | v38.79,12.88 39.7,12.88 40.46,13.64 40.46,22.17 41.83,23.55 | U8.1 46.56,15.8 46.56,15.77 v45.49,15.77
CPU_R/W'  (via drill 0.2)
  Top 0.152: U3.3 25.22,30.56 v23.55,30.56
  Bottom 0.152: RS1.R4B 10.29,15.93 10.29,16.38 10.59,16.69 12.12,16.69 12.73,17.3 13.95,17.3 14.4,17.75 14.4,21.87 14.86,22.33 16.54,22.33 16.99,22.78 16.99,26.59 17.6,27.2 21.11,27.2 23.55,29.64 v23.55,30.56
CPU_RESET*  (via drill 0.2)
  Top 0.152: U5.2 25.25,10.74 v22.78,10.74 | U5.6 25.25,15.93 v23.24,15.93 | J8.3 6.48,4.95 10.9,4.95 12.73,6.78 v23.09,6.78 23.7,6.78 24,7.09 27.81,7.09 29.34,5.56 33.91,5.56 34.82,4.65 38.48,4.65 39.09,5.26 39.09,7.09 39.85,7.85 39.85,9.07 41.53,10.74 42.49,10.74 68B09E.37
  Bottom 0.152: v23.24,15.93 22.63,15.32 22.63,14.1 23.24,13.49 23.24,11.2 v22.78,10.74 22.78,8 23.09,7.7 v23.09,6.78
CPU_TSC  (via drill 0.2)
  Top 0.152: v77.19,12.12 77.19,12.57 76.58,13.18 73.69,13.18 73.23,13.64 70.03,13.64 69.42,14.25 65.46,14.25 64.85,14.86 56.46,14.86 56.01,14.4 54.03,14.4 53.11,13.49 50.67,13.49 50.22,13.95 v45.03,13.95
  Bottom 0.152: 44.27,5.71 45.03,5.71 45.64,5.1 45.64,4.04 45.8,3.89 47.02,3.89 U1.2 47.17,3.89 | 68B09E.39 44.27,5.71 | v77.19,12.12 78.56,12.12 78.87,11.81 78.87,9.68 79.17,9.37 79.17,6.02 79.48,5.71 TGT_HDR.39 80.7,5.71 | U14.4 47.02,45.64 44.73,45.64 44.27,45.19 44.27,34.37 45.34,33.3 45.34,32.54 44.58,31.77 44.58,28.12 45.64,27.05 45.64,24.31 45.34,24 45.34,20.65 44.73,20.04 44.73,17.6 44.42,17.3 44.42,15.16 45.03,14.55 v45.03,13.95 45.03,13.34 45.34,13.03 45.34,10.59 44.27,9.53 44.27,5.71
CPU_TSC'  (via drill 0.2)
  Top 0.152: 36.8,9.53 37.11,9.53 | v35.59,7.85 36.5,7.85 36.8,8.15 36.8,9.53 | 36.8,9.53 U7.1
  Bottom 0.152: v35.59,7.85 34.21,6.48 34.21,2.06 34.67,1.6 50.67,1.6 51.59,2.51 53.21,2.51 U1.16
D0  (via drill 0.2)
  Top 0.152: 62.85,30.54 U12.18 | 62.85,30.54 62.84,30.56 | U4.11 29.82,39.39 37.41,39.39 v37.72,39.7 | 68B09E.31 42.6,25.98 51.89,25.98 53.87,27.96 55.55,27.96 56.31,27.2 58.9,27.2 59.66,26.44 61.04,26.44 61.8,27.2 65,27.2 65.3,27.51 65.3,29.64 64.54,30.4 62.71,30.4 62.85,30.54
  Bottom 0.152: v37.72,39.7 38.79,38.63 38.79,31.32 40.77,29.34 40.77,27.2 41.99,25.98 42.44,25.98 42.49,26.04 68B09E.31
D1  (via drill 0.2)
  Top 0.152: U4.12 29.82,40.62 31.17,40.62 31.47,40.31 38.02,40.31 v38.63,39.7 | 68B09E.30 48.39,28.57 49.3,29.49 49.3,31.47 49.76,31.93 49.76,33.76 50.22,34.21 54.18,34.21 56.01,32.38 56.01,30.4 56.31,30.1 59.05,30.1 60.73,31.77 62.89,31.77 U12.17
  Bottom 0.152: v38.63,39.7 39.09,39.24 39.09,31.47 41.99,28.57 68B09E.30
D2  (via drill 0.2)
  Top 0.152: U12.16 62.89,32.99 60.68,32.99 60.07,32.38 56.46,32.38 54.33,34.52 50.06,34.52 49.45,33.91 49.45,32.08 49,31.62 46.1,31.62 45.8,31.93 44.88,31.93 44.12,31.17 42.6,31.17 68B09E.29 | U4.13 29.87,41.99 31.77,41.99 32.23,42.44 v38.18,42.44
  Bottom 0.152: v38.18,42.44 39.39,41.22 39.39,33.45 41.68,31.17 42.44,31.17 68B09E.29
D3  (via drill 0.2)
  Top 0.152: 42.6,33.6 45.64,33.6 46.86,34.82 54.48,34.82 56.62,32.69 59.92,32.69 61.59,34.37 62.84,34.37 U12.15 | 68B09E.28 42.6,33.6 | 42.6,33.6 42.44,33.6 | U4.14 29.82,43.2 38.94,43.2 v39.24,42.9
  Bottom 0.152: v39.24,42.9 39.7,42.44 39.7,34.98 41.07,33.6 42.6,33.6 68B09E.28
D4  (via drill 0.2)
  Top 0.152: 68B09E.27 45.19,36.2 46.86,37.87 53.42,37.87 54.03,37.26 59.92,37.26 61.59,35.59 62.89,35.59 U12.14 | U4.15 30.12,44.45 30.4,44.42 31.17,44.42 31.93,43.66 35.13,43.66 35.89,44.42 38.02,44.42 v38.33,44.12
  Bottom 0.152: v38.33,44.12 38.94,43.51 39.55,43.51 40,43.05 40,37.11 40.92,36.2 68B09E.27 42.6,36.2
D5  (via drill 0.2)
  Top 0.152: 68B09E.26 42.85,38.73 42.9,38.79 43.2,38.79 43.81,38.18 53.57,38.18 54.18,37.57 60.22,37.57 60.98,36.8 62.89,36.8 U12.13 | U4.16 29.87,45.64 31.62,45.64 31.93,45.34 v37.57,45.34
  Bottom 0.152: v37.57,45.34 39.39,45.34 39.7,45.03 39.7,43.81 40.31,43.2 40.31,39.24 40.77,38.79 42.6,38.79 68B09E.26
D6  (via drill 0.2)
  Top 0.152: U4.17 29.79,47.02 32.54,47.02 33.76,48.23 v39.39,48.23 | 68B09E.25 42.7,41.27 42.75,41.22 44.12,41.22 45.03,42.14 50.52,42.14 52.35,40.31 53.72,40.31 54.79,39.24 56.01,39.24 56.62,39.85 59.92,39.85 61.59,38.18 62.97,38.18 62.97,38.15 U12.12
  Bottom 0.152: v39.39,48.23 40,47.62 40,43.97 40.62,43.36 40.62,41.53 40.92,41.22 42.44,41.22 42.49,41.27 68B09E.25
D7  (via drill 0.2)
  Top 0.152: U4.18 29.82,48.23 32.38,48.23 33.76,49.61 34.82,49.61 35.28,49.15 39.85,49.15 v40.31,49.61 | 68B09E.24 43.2,43.81 44.88,45.49 53.26,45.49 54.33,44.42 54.33,40.16 54.94,39.55 55.85,39.55 56.46,40.16 60.07,40.16 60.98,39.24 62.81,39.24 62.81,39.27 U12.11
  Bottom 0.152: v40.31,49.61 40.31,44.12 40.62,43.81 68B09E.24 42.6,43.81
EM_D_DIR  (via drill 0.2)
  Top 0.152: U4.1 21.44,50.8 22.63,49.61 26.59,49.61 v27.05,50.06 | v54.79,19.74 52.05,19.74 51.59,20.19 46.41,20.19 46.1,20.5 44.73,20.5 44.12,19.89 39.39,19.89 39.24,20.04 36.04,20.04 34.82,18.82 30.1,18.82 29.64,19.28 29.64,19.89 28.12,21.41 v26.9,21.41
  Bottom 0.152: v27.05,50.06 26.75,49.76 26.75,42.6 25.83,41.68 25.83,27.66 26.9,26.59 v26.9,21.41 | U8.11 53.01,19.68 52.96,19.74 v54.79,19.74
EM_D_EN*  (via drill 0.2)
  Top 0.152: U4.19 29.72,49.61 28.42,49.61 v27.96,50.06 | v27.51,45.34 27.2,45.03 27.2,42.75 27.96,41.99 27.96,39.09 28.42,38.63 34.21,38.63 34.67,39.09 39.09,39.09 39.85,38.33 39.85,36.04 40.77,35.13 v45.34,35.13 45.34,35.89 46.71,37.26 v51.44,37.26
  Bottom 0.152: v27.51,45.34 27.51,49.61 v27.96,50.06 | 47.14,35.13 47.17,34.98 | 47.14,35.13 U2.6 | v45.34,35.13 47.14,35.13 | U2.9 53.19,35.13 53.19,34.9 53.26,34.82 54.48,34.82 54.79,35.13 54.79,36.8 54.33,37.26 v51.44,37.26
EM_OVERRIDE_INTS  (via drill 0.2)
  Top 0.152: J7.28 14.4,35.13 16.69,35.13 16.99,35.43 16.99,36.65 18.36,38.02 20.04,38.02 21.26,36.8 21.87,36.8 23.39,38.33 24.77,38.33 v25.22,38.79 26.9,38.79 28.27,37.41 35.43,37.41 36.35,38.33 37.26,38.33 37.57,38.02 37.57,37.57 37.87,37.26 38.18,37.26 38.48,36.96 38.48,32.23 41.07,29.64 v45.19,29.64 | U17.10 62.25,20.95 62.1,21.11 v63.93,21.11 60.73,21.11 59.82,22.02 54.63,22.02 53.72,21.11 v49.61,21.11 | v63.93,17.3 63.02,17.3 62.86,17.14 U17.13 63.02,17.14 63.17,17.3 v63.93,17.3 | v63.93,17.3 67.59,17.3 67.74,17.14 U17.2
  Bottom 0.152: v63.93,21.11 v63.93,17.3 | U10.1 19.2,18.36 20.34,18.36 21.11,17.6 21.72,17.6 22.02,17.91 22.02,18.82 20.95,19.89 20.95,21.41 22.63,23.09 22.63,25.22 25.22,27.81 v25.22,38.79 | v49.61,21.11 49.91,21.41 49.91,25.83 50.52,26.44 50.52,27.81 49.61,28.73 47.47,28.73 47.17,28.57 U2.1 47.09,28.65 47.02,28.73 45.49,28.73 45.19,29.03 v45.19,29.64
EN_ADDR_TO_TGT*  (via drill 0.2)
  Top 0.152: U20.15 62.74,43.18 62.76,43.2 v64.39,43.2 65.3,43.2 66.06,42.44 66.06,40.62 66.83,39.85 68.35,39.85 70.94,42.44 74.14,42.44 v74.6,41.99 | U22.15 62.94,3.81 63.17,4.04 64.85,4.04 65.61,4.8 65.61,12.73 | 65.61,12.73 67.28,12.73 67.59,12.42 69.11,12.42 69.72,13.03 72.92,13.03 73.84,12.12 v75.97,12.12 | U7.3 36.93,11.96 38.33,11.96 38.79,11.51 v38.79,10.74 | v40.77,12.12 45.19,12.12 46.1,13.03 48.23,13.03 49.61,11.66 54.63,11.66 54.94,11.96 59.05,11.96 59.82,12.73 59.82,13.34 60.12,13.64 64.24,13.64 65.15,12.73 65.61,12.73
  Bottom 0.152: 74.14,30.56 74.14,27.81 75.21,26.75 75.21,16.08 75.97,15.32 | 74.14,30.56 75.67,30.56 75.82,30.71 76.05,30.48 U21.15 76.1,30.56 74.14,30.56 | 74.14,30.56 74.14,41.53 v74.6,41.99 77.19,41.99 77.27,41.91 U19.15 | v75.97,12.12 75.97,15.32 | U11.15 77.29,15.32 75.97,15.32 | v38.79,10.74 40,10.74 40.77,11.51 v40.77,12.12 | U2.11 53.87,32.38 54.03,32.54 54.63,32.54 55.4,33.3 55.4,35.43 55.7,35.74 55.7,39.39 56.46,40.16 58.9,40.16 60.12,41.38 60.12,42.6 60.73,43.2 v64.39,43.2
GND  (via drill 0.2)
  Top 0.152: 68.43,23.55 69.72,23.55 69.88,23.39 69.88,20.95 | 69.88,20.95 69.88,19.89 69.72,19.74 68.43,19.74 U17.4 | 69.88,20.95 U17.5 | U3.15 19.18,29.18 v21.41,29.18 | U3.1 25.27,28.12 v23.7,28.12 | U7.9 30.63,15.93 29.18,15.93 v28.88,16.23 28.88,15.01 29.18,14.71 30.68,14.71 U7.10
  Top 0.406: v21.41,39.39 19.89,39.39 U4.10 | U20.8 68.5,50.82 70.18,50.82 70.48,50.52 v71.09,50.52 71.86,49.76 71.86,49.15 71.75,49.05 C10.2 | U12.10 72.95,39.39 v70.48,39.39 | U17.7 68.43,23.55 69.11,23.55 v69.11,24.46 | U22.8 68.55,11.51 70.64,11.51 | U3.8 25.27,36.8 v26.9,36.8 | U6.7 36.98,36.2 v35.43,36.2 | U7.7 v38.33,17.14 | U5.11 21.11,13.34 v21.56,13.79 | C4.2 76.86,36.32 76.89,36.35 v78.11,36.35 | C3.2 71.7,17.91 71.86,18.06 v73.08,18.06 | C17.2 71.12,11.02 70.64,11.51 | 70.64,11.51 v70.64,11.81 | C8.2 19.46,4.34 18.67,4.34 v18.06,3.73 | v51.44,7.09 C16.2 | C18.2 51.13,43.36 51.28,42.9 v51.28,42.29
  Top 0.508: C1.- 77.5,3.83 77.5,4.5 v79.17,4.5
  Bottom 0.152: U11.1 71.2,13.95 70.64,13.95 v70.64,11.81 | U16.19 29.82,5.1 v27.51,5.1 | U13_PIGGY.13 77.32,4.5 76.12,4.5 | 75.97,5.71 U13_PIGGY.12 | 75.97,5.71 75.97,8 76.12,8.15 77.27,8.15 U13_PIGGY.10 77.47,8.15 78.56,8.15 78.72,8.31 78.72,9.22 78.56,9.37 77.52,9.37 U13_PIGGY.9 | U14.10 53.16,49.45 v51.59,49.45 | U14.12 53.21,47.17 v51.59,47.17 | U14.14 53.21,44.27 51.74,44.27 51.28,43.81 51.28,43.2 | U14.15 53.21,43.2 51.28,43.2 | v51.28,42.29 51.28,43.2 | U14.1 47.17,41.99 45.8,41.99 45.49,42.29 v45.49,43.2 47.12,43.2 U14.2 | U10.11 25.2,22.33 24.61,22.33 24.46,22.02 v22.78,22.02 22.78,22.48 23.7,23.39 | U10.10 25.2,23.39 23.7,23.39 | U10.9 24,24.77 23.7,24.46 23.7,23.39 | U13.9 25.25,50.37 v23.55,50.37 | U9.9 v38.33,24.77 38.33,23.85 38.02,23.55 36.78,23.55 U9.10 | U15.19 29.87,30.4 v28.12,30.4 | U9.13 36.78,19.58 36.93,19.74 37.87,19.74 38.33,20.19 v38.33,21.11 36.65,21.11 U9.12 | U2.2 47.19,29.79 v48.69,29.79 48.69,31.01 48.54,31.17 47.14,31.17 U2.3 | 75.97,5.71 75.97,4.65 76.12,4.5 | 76.12,4.5 v79.17,4.5
  Bottom 0.406: U16.10 19.81,15.32 v21.56,15.32 | U19.8 71.09,49.66 v71.09,50.52 68.2,50.52 68.05,50.37 68.05,49.76 C7.2 | v70.48,39.39 70.48,38.18 70.03,38.18 U21.8 69.88,38.18 68.15,38.18 C5.2 | U11.8 71.14,22.94 69.72,22.94 69.11,23.55 v69.11,24.46 | U13_PIGGY.7 71.12,10.9 70.64,10.9 | v70.64,11.81 70.64,10.9 | U14.8 47.12,50.77 v48.69,50.77 | U1.12 53.16,7.54 53.01,7.7 52.05,7.7 v51.44,7.09 | U15.10 19.76,40.62 v21.41,40.62 | U10.7 19.25,26.14 v20.8,26.14 | U15.1 19.76,29.18 v21.41,29.18 | v18.06,3.73 19.13,3.73 U16.1 | 47.02,36.2 v48.69,36.2 | 47.02,36.2 U2.7 47.02,36.27 47.02,36.2 | U13.7 22.02,51.44 v22.48,50.98 | U9.7 30.48,26.14 29.03,26.14 v28.73,26.44 | C21.2 61.65,49.61 v64.69,49.61 | C6.2 47.02,37.95 47.02,36.2 | C14.2 36.8,33.81 36.8,35.59 36.2,36.2 v35.43,36.2 | C11.2 36.83,16.71 37.26,17.14 v38.33,17.14 | 70.64,10.9 70.64,10.74 69.39,10.74 C20.2 | C19.2 61.8,11.48 61.8,10.74 61.34,10.29 v60.58,10.29 | U8.7 47.73,23.49 47.78,23.55 v48.69,23.55 | C9.2 61.49,18.52 61.49,19.13 61.19,19.43 v60.73,19.43 | C15.2 35.43,50.75 v35.43,49.91
  Bottom 0.508: C2.- 31.23,44.42 v32.99,44.42
  pour gnd (isolate 0.254, rank 2): 69.85,53.98 71.12,52.7 83.82,52.7 84.45,52.07 84.45,2.54 83.82,1.91 71.12,1.91 69.85,0.64 1.27,0.64 0.64,1.27 0.64,53.34 1.27,53.98 31.75,53.98 32.38,53.34 32.38,52.07 33.02,51.44 40,51.44 40.64,52.07 40.64,53.34 41.27,53.98
J8_13  (via drill 0.2)
  Top 0.152: J8.13 5.71,18.36 7.54,16.54 9.22,16.54 9.98,17.3 16.38,17.3 18.36,19.28 24,19.28 25.07,18.21 27.81,18.21 28.12,18.52 34.98,18.52 36.2,19.74 39.09,19.74 39.24,19.58 44.27,19.58 44.58,19.89 v45.49,19.89 51.44,19.89 52.81,18.52 v54.79,18.52
  Bottom 0.152: U8.4 47.12,19.68 47.17,19.58 46.71,19.89 v45.49,19.89 | U8.12 53.49,18.52 v54.79,18.52
N$2
  Bottom 0.152: RS1.R1A 8.76,13.37 8.46,13.34 7.54,13.34 7.09,12.88 7.09,11.35 6.93,11.2 6.93,9.37 5.87,8.31 5.71,8.31 J8.5
N$3
  Bottom 0.152: 8.68,14.25 RS1.R2A 8.62,14.25 7.7,14.25 6.78,13.34 6.78,11.81 5.87,10.9 5.82,10.9 J8.7
N$4
  Bottom 0.152: RS1.R3A 7.85,15.01 6.93,15.93 6.93,19.89 5.87,20.95 J8.15
N$5
  Bottom 0.152: RS1.R4A 8.69,15.77 7.85,15.77 7.24,16.38 7.24,20.04 6.93,20.34 6.93,24.92 6.02,25.83 5.71,25.98 J8.19
N$6
  Bottom 0.152: J8.17 4.5,24.71 4.5,26.9 4.95,27.36 6.17,27.36 7.39,28.57 8.76,28.57 8.76,28.61 RS3.R1A
N$7
  Bottom 0.152: RS3.R2A 8.68,29.49 6.63,29.49 J8.21
N$8
  Bottom 0.152: J8.23 5.82,31.17 5.71,31.17 6.63,30.25 RS3.R3A | RS3.R3A 8.76,30.25 | RS3.R3A
N$9
  Bottom 0.152: J8.25 5.77,33.66 7.09,34.98 7.09,38.48 7.39,38.79 8.61,38.79 8.63,38.8 RS2.R1A
N$10
  Bottom 0.152: J8.27 6.78,37.26 6.78,39.09 7.24,39.55 8.61,39.55 8.67,39.6 RS2.R2A
N$11
  Bottom 0.152: J8.29 5.71,38.79 7.39,40.46 8.61,40.46 8.67,40.41 RS2.R3A
N$12
  Bottom 0.152: RS2.R4A 8.63,41.2 8.56,41.27 J8.31
N$13
  Bottom 0.152: RS4.R1A 8.73,43.32 8.15,42.75 6.78,42.75 J8.33
N$14  (via drill 0.2)
  Top 0.152: v7.54,43.51 6.78,42.75 5.1,42.75 4.5,43.36 4.5,45.19 J8.35
  Bottom 0.152: RS4.R2A 8.11,44.69 7.54,44.12 v7.54,43.51
N$15  (via drill 0.2)
  Top 0.152: v7.24,44.88 6.78,45.34 6.78,47.78 5.71,48.84 J8.37
  Bottom 0.152: RS4.R3A 7.84,45.48 v7.24,44.88
N$16
  Bottom 0.152: RS4.R4A 7.36,46.28 6.33,45.19 4.95,45.19 4.5,45.64 4.5,50.22 J8.39
N$17  (via drill 0.2)
  Top 0.152: v10.13,37.87 10.13,38.94 11.05,39.85 16.84,39.85 17.6,40.62 19.74,40.62 U4.9
  Bottom 0.152: RS2.R1B 10.13,38.77 v10.13,37.87
N$18  (via drill 0.2)
  Top 0.152: v11.51,38.02 10.59,37.11 9.68,37.11 9.37,37.41 9.37,38.63 10.9,40.16 16.69,40.16 17.14,40.62 17.14,41.53 17.45,41.83 19.66,41.83 U4.8
  Bottom 0.152: RS2.R2B 10.38,39.55 11.2,39.55 11.51,39.24 v11.51,38.02
N$19  (via drill 0.2)
  Top 0.152: v11.51,41.68 12.27,42.44 16.84,42.44 17.45,43.05 19.43,43.05 19.58,43.2 19.61,43.18 U4.7
  Bottom 0.152: RS2.R3B 11.3,40.41 11.51,40.62 v11.51,41.68
N$20  (via drill 0.2)
  Top 0.152: v8.76,42.14 10.9,42.14 11.51,42.75 16.69,42.75 16.99,43.05 16.99,43.97 17.45,44.42 19.58,44.42 19.61,44.45 U4.6
  Bottom 0.152: v8.76,42.14 9.98,42.14 10.29,41.83 10.29,41.22 10.31,41.2 RS2.R4B
N$21  (via drill 0.2)
  Top 0.152: v9.53,42.9 9.53,43.51 9.98,43.97 11.81,43.97 12.88,45.03 16.84,45.03 17.45,45.64 19.66,45.64 U4.5
  Bottom 0.152: v9.53,42.9 10.13,42.9 10.29,43.05 10.29,43.77 RS4.R1B
N$22  (via drill 0.2)
  Top 0.152: v11.51,44.73 12.12,45.34 16.69,45.34 16.99,45.64 16.99,46.71 17.3,47.02 19.71,47.02 U4.4
  Bottom 0.152: RS4.R2B 10.37,44.73 v11.51,44.73
N$23  (via drill 0.2)
  Top 0.152: v11.51,46.41 11.51,47.02 11.96,47.47 16.84,47.47 17.6,48.23 19.28,48.23 19.3,48.26 U4.3
  Bottom 0.152: RS4.R3B 11.35,45.48 11.51,45.64 v11.51,46.41
N$24  (via drill 0.2)
  Top 0.152: U4.2 19.66,49.53 19.58,49.45 17.3,49.45 16.99,49.15 16.99,48.08 16.69,47.78 11.81,47.78 11.2,47.17 v10.44,47.17
  Bottom 0.152: RS4.R4B 10.44,46.4 v10.44,47.17
N$25
  Bottom 1.27: IC2.8 IC1.8
N$26
  Bottom 1.27: IC2.9 IC1.9
N$27
  Bottom 1.27: IC2.10 IC1.10
N$28
  Bottom 1.27: IC2.11 IC1.11
N$29
  Bottom 1.27: IC2.12 IC1.12
N$30
  Bottom 1.27: IC2.13 IC1.13
N$31
  Bottom 1.27: IC2.14 IC1.14
N$32
  Bottom 1.27: IC2.15 IC1.15
N$33
  Bottom 1.27: IC2.16 IC1.16
N$34
  Bottom 1.27: IC2.17 IC1.17
N$35
  Bottom 1.27: IC2.18 IC1.18
N$36
  Bottom 1.27: IC2.19 IC1.19
N$37
  Bottom 1.27: IC2.20 IC1.20
N$38
  Bottom 1.27: IC1.21 IC2.21
N$39
  Bottom 1.27: IC1.22 IC2.22
N$40
  Bottom 1.27: IC1.23 IC2.23
N$41
  Bottom 1.27: IC1.31 IC2.31
N$42
  Bottom 1.27: IC1.30 IC2.30
N$43
  Bottom 1.27: IC1.29 IC2.29
N$44
  Bottom 1.27: IC1.28 IC2.28
N$45  (via drill 0.2)
  Top 0.152: v54.79,17.3 53.57,17.3 51.74,19.13 v49,19.13
  Bottom 0.152: U8.3 47.14,18.36 48.39,18.36 49,18.97 v49,19.13 | U8.13 53.24,17.3 v54.79,17.3
N$46  (via drill 0.2)
  Top 0.152: v45.95,27.66 47.93,27.66 49.61,29.34 49.61,31.32 50.98,32.69 v50.98,33.45
  Bottom 0.152: U8.5 45.8,20.95 45.64,21.11 45.64,23.85 45.95,24.15 v45.95,27.66 | v50.98,33.45 50.67,33.76 50.67,35.89 51.13,36.35 53.11,36.35 53.24,36.22 U2.8
N$47
  Bottom 1.27: IC1.27 IC2.27
N$48
  Bottom 1.27: IC1.26 IC2.26
N$49
  Bottom 1.27: IC1.25 IC2.25
N$50
  Bottom 1.27: IC1.24 IC2.24
N$51
  Bottom 1.27: IC1.38 IC2.38
N$52
  Bottom 1.27: IC1.36 IC2.36
N$53
  Bottom 1.27: IC1.33 IC2.33
N$54
  Bottom 1.27: IC2.6 IC1.6
N$55
  Bottom 1.27: IC2.5 IC1.5
N$56
  Bottom 1.27: IC1.32 IC2.32
N$57
  Bottom 1.27: IC1.39 IC2.39
N$58
  Bottom 1.27: IC1.37 IC2.37
N$59
  Bottom 1.27: IC2.2 IC1.2
N$60
  Bottom 1.27: IC1.40 IC2.40
N$61  (via drill 0.2)
  Top 0.152: J7.3 15.77,5.71 15.77,5.56 14.71,4.5 12.57,4.5 12.12,4.04 12.12,2.82 11.81,2.51 v7.7,2.51
  Bottom 0.152: RS10.R3B 8,4.04 7.7,3.73 v7.7,2.51
N$62  (via drill 0.2)
  Top 0.152: v7.39,6.93 9.37,6.93 9.98,6.33 11.81,6.33 12.57,7.09 14.71,7.09 J7.5
  Bottom 0.152: RS10.R2B 8.62,4.95 7.7,4.95 7.39,5.26 v7.39,6.93
N$63
  Bottom 1.27: IC2.3 IC1.3
N$64
  Bottom 1.27: IC2.4 IC1.4
N$65
  Bottom 1.27: IC1.34 IC2.34
N$66
  Bottom 1.27: IC1.35 IC2.35
N$67
  Bottom 1.27: IC2.7 IC1.7
N$68
  Bottom 1.27: IC2.1 IC1.1
N$81  (via drill 0.2)
  Top 0.152: v7.39,8.15 9.22,8.15 9.68,8.61 9.68,10.44 10.9,11.66 v11.96,11.66
  Bottom 0.152: RS13.R3B 8.67,9.07 7.7,9.07 7.39,8.76 v7.39,8.15 | v11.96,11.66 12.57,12.27 14.86,12.27 15.77,13.18 15.77,13.23 J7.9
N$82  (via drill 0.2)
  Top 0.152: J7.11 14.71,14.71 12.88,14.71 11.96,15.62 9.68,15.62 8.15,14.1 8.15,12.57 8.61,12.12 8.61,10.9 v7.7,9.98
  Bottom 0.152: RS13.R2B 8.67,9.98 v7.7,9.98
N$83  (via drill 0.2)
  Top 0.152: v8.15,17.3 8.15,19.13 9.22,20.19 11.51,20.19 12.27,20.95 12.27,21.72 12.57,22.02 14.86,22.02 15.77,21.11 15.93,21.11 15.93,21.01 J7.15
  Bottom 0.152: RS9.R3B 8,19.28 7.7,18.97 7.7,17.75 v8.15,17.3
N$84
  Bottom 0.152: RS9.R2B 8.68,20.04 8,20.04 7.7,20.34 7.7,21.26 9.37,22.94 11.05,22.94 12.73,24.61 14.71,24.61 15.77,23.55 15.82,23.55 J7.17
N$85  (via drill 0.2)
  Top 0.152: v7.7,24.46 7.7,25.68 8.46,26.44 10.13,26.44 11.2,27.51 14.86,27.51 15.93,28.57 J7.21
  Bottom 0.152: RS12.R3B 8.63,24.46 v7.7,24.46
N$86  (via drill 0.2)
  Top 0.152: v7.7,26.75 9.98,26.75 11.2,27.96 11.2,29.03 12.12,29.95 14.71,29.95 J7.23
  Bottom 0.152: RS12.R2B 7.91,25.16 7.7,25.38 v7.7,26.75
N$87
  Bottom 0.152: RS11.R3B 7.24,49.76 6.78,49.3 6.78,47.62 7.39,47.02 9.22,47.02 10.13,47.93 10.74,47.93 11.2,47.47 14.71,47.47 15.77,46.41 15.82,46.41 J7.35
N$88  (via drill 0.2)
  Top 0.152: v8.76,52.2 12.42,52.2 12.73,52.5 14.86,52.5 15.93,51.44 J7.39
  Bottom 0.152: RS11.R1B 8.66,51.44 8.76,51.44 v8.76,52.2
N$89
  Bottom 0.152: RS10.R4B 8.76,3.21 8.76,2.82 9.07,2.51 12.73,2.51 13.34,3.12 J7.2
N$90
  Bottom 0.152: RS10.R1B 8.73,6.13 8.92,6.33 11.35,6.33 13.34,8.31 J7.6
N$91  (via drill 0.2)
  Top 0.152: v10.29,7.24 11.66,7.24 12.12,7.7 12.12,8.61 13.34,9.83 J7.8
  Bottom 0.152: RS13.R4B 8.76,8.29 8.76,7.54 9.07,7.24 v10.29,7.24
N$92  (via drill 0.2)
  Top 0.152: J7.12 13.34,15.93 9.53,15.93 7.85,14.25 v7.85,11.81
  Bottom 0.152: 8.71,10.74 RS13.R1B | 8.71,10.74 8.76,10.74 | 8.71,10.74 8.15,10.74 7.85,11.05 v7.85,11.81
N$93
  Bottom 0.152: RS9.R1B 8.61,20.92 8.61,21.72 9.53,22.63 11.2,22.63 12.12,23.55 13.34,23.55 J7.18
N$94
  Bottom 0.152: RS9.R4B 8.76,18.45 8.76,17.91 9.37,17.3 12.12,17.3 13.18,18.36 13.34,18.36 J7.14
N$95  (via drill 0.2)
  Top 0.152: v7.7,22.78 8.61,23.7 8.61,25.53 9.07,25.98 13.28,25.98 J7.20
  Bottom 0.152: RS12.R4B 8.61,23.45 8.52,23.55 7.85,23.55 7.7,23.39 v7.7,22.78
N$96
  Bottom 0.152: RS12.R1B 8.73,26.71 9.07,27.05 10.29,27.05 11.2,27.96 11.2,29.03 13.34,31.17 J7.24
N$97  (via drill 0.2)
  Top 0.152: v8.46,36.96 8.92,36.5 10.59,36.5 11.05,36.96 11.51,36.96 13.34,38.79 J7.30
  Bottom 0.152: RS8.R4A 8.46,36.12 v8.46,36.96
N$98
  Bottom 0.152: RS8.R1A 8.69,33.76 8,33.76 7.7,34.06 7.7,37.26 8.15,37.72 9.07,37.72 9.68,37.11 11.66,37.11 12.27,37.72 12.27,42.75 J7.34
N$99  (via drill 0.2)
  Top 0.152: v8.76,48.08 8.76,46.1 9.22,45.64 12.57,45.64 13.34,46.41 J7.36
  Bottom 0.152: RS11.R4B 8.76,48.96 v8.76,48.08
N$100  (via drill 0.2)
  Top 0.152: v7.54,48.08 v7.54,50.52
  Bottom 0.152: J7.38 12.22,47.78 11.35,47.78 10.9,48.23 9.98,48.23 9.07,47.32 8.31,47.32 v7.54,48.08 | RS11.R2B 8.66,50.56 8.61,50.52 v7.54,50.52
N$101
  Bottom 0.152: RS10.R4A 10.34,3.23 11.76,3.23 12.88,4.34 13.95,4.34 14.4,3.89 14.4,2.51 15.16,1.75 31.01,1.75 31.77,2.51 31.77,13.18 31.01,13.95 29.79,13.95 U16.12
N$102
  Bottom 0.152: U16.14 29.79,11.51 31.17,11.51 31.47,11.2 31.47,2.67 30.86,2.06 15.47,2.06 14.71,2.82 14.71,4.04 14.1,4.65 12.73,4.65 12.12,4.04 RS10.R3A
N$103
  Bottom 0.152: RS10.R2A 10.38,4.9 11.76,4.9 12.12,5.26 12.12,6.17 12.73,6.78 16.54,6.78 16.99,6.33 16.99,2.97 17.45,2.51 30.71,2.51 31.17,2.97 31.17,8.76 31.01,8.92 29.79,8.92 U16.16
N$104
  Bottom 0.152: RS10.R1A 10.34,5.66 11.46,5.66 11.81,6.02 11.81,6.33 12.57,7.09 16.84,7.09 17.3,6.63 17.3,3.12 17.6,2.82 26.44,2.82 26.75,3.12 26.75,6.02 27.05,6.33 29.82,6.33 U16.18
N$105
  Bottom 0.152: U16.3 19.71,6.33 18.21,6.33 17.3,7.24 17.3,8.46 16.38,9.37 12.42,9.37 11.35,8.31 10.34,8.31 RS13.R4A
N$106
  Bottom 0.152: U16.5 19.71,8.92 17.3,8.92 16.54,9.68 12.27,9.68 11.81,9.22 10.42,9.22 RS13.R3A
N$107
  Bottom 0.152: U16.7 19.66,11.35 18.36,11.35 18.06,11.66 18.06,13.34 16.99,14.4 12.88,14.4 12.12,13.64 12.12,13.03 11.2,12.12 11.2,10.13 11.05,9.98 10.57,9.98 RS13.R2A
N$108
  Bottom 0.152: U16.9 19.71,13.95 17.91,13.95 17.14,14.71 12.73,14.71 11.81,13.79 11.81,13.18 10.29,11.66 10.29,10.74 10.34,10.74 RS13.R1A
N$109  (via drill 0.2)
  Top 0.152: v11.51,18.06 12.27,18.82 12.27,19.28 12.57,19.58 26.29,19.58 v27.05,18.82
  Bottom 0.152: RS9.R4A 10.36,18.52 11.05,18.52 v11.51,18.06 | U15.12 29.79,39.39 28.42,39.39 27.81,38.79 27.81,34.98 26.29,33.45 26.29,27.66 27.2,26.75 27.2,22.17 27.66,21.72 27.66,20.95 27.36,20.65 27.05,20.65 26.75,20.34 26.75,19.13 v27.05,18.82
N$110  (via drill 0.2)
  Top 0.152: v11.51,19.28 12.12,19.89 v27.36,19.89
  Bottom 0.152: RS9.R3A v11.51,19.28 | v27.36,19.89 27.96,20.5 27.96,21.87 27.51,22.33 27.51,26.9 26.59,27.81 26.59,33.3 28.12,34.82 28.12,36.5 28.42,36.8 29.82,36.8 U15.14
N$111  (via drill 0.2)
  Top 0.152: v11.51,21.26 11.51,23.39 12.73,24.61 16.54,24.61 17.3,23.85 21.87,23.85 22.33,23.39 32.23,23.39 v33.15,24.31
  Bottom 0.152: RS9.R2A 11.25,20.08 11.51,20.34 v11.51,21.26 | v33.15,24.31 33.45,24.61 33.45,33.15 32.23,34.37 29.79,34.37 29.87,34.29 U15.16
N$112  (via drill 0.2)
  Top 0.152: v10.59,21.87 11.2,22.63 11.2,23.55 12.57,24.92 16.69,24.92 17.45,24.15 22.02,24.15 22.48,23.7 31.17,23.7 v32.84,25.38
  Bottom 0.152: RS9.R1A 10.59,21.15 v10.59,21.87 | U15.18 29.77,31.62 27.66,31.62 27.2,31.17 27.2,28.12 27.81,27.51 31.62,27.51 32.84,26.29 v32.84,25.38
N$113
  Bottom 0.152: RS12.R4A 10.34,23.55 11.05,23.55 11.81,24.31 11.81,26.75 12.27,27.2 17.14,27.2 18.21,28.27 18.21,31.47 18.52,31.77 19.71,31.77 U15.3
N$114
  Bottom 0.152: RS12.R3A 10.42,24.46 11.05,24.46 11.51,24.92 11.51,26.9 12.12,27.51 16.99,27.51 17.91,28.42 17.91,33.91 18.21,34.21 19.66,34.21 U15.5
N$115
  Bottom 0.152: RS12.R2A 10.38,25.22 11.05,25.22 11.2,25.38 11.2,27.05 11.81,27.66 11.81,28.73 12.73,29.64 16.84,29.64 17.6,30.4 17.6,36.5 17.91,36.8 19.61,36.8 U15.7
N$116
  Bottom 0.152: RS12.R1A 10.29,26 10.29,26.59 11.51,27.81 11.51,28.88 12.57,29.95 16.69,29.95 17.3,30.56 17.3,39.09 17.6,39.39 19.71,39.39 U15.9
N$117  (via drill 0.2)
  Top 0.152: v22.48,45.64 22.48,42.9 23.09,42.29 27.2,42.29 27.66,41.83 27.66,38.94 28.27,38.33 34.37,38.33 34.82,38.79 38.94,38.79 39.55,38.18 39.55,35.89 40.62,34.82 44.12,34.82 44.58,34.37 45.95,34.37 46.71,35.13 49.91,35.13 51.13,36.35 55.4,36.35 56.62,35.13 59.36,35.13 59.66,35.43 v60.43,35.43 | v66.06,35.89 66.06,28.88 66.52,28.42 v67.89,28.42
  Bottom 0.152: U13_PIGGY.1 71.25,3.15 71.25,3.12 72.92,3.12 73.84,4.04 73.84,5.1 73.08,5.87 73.08,6.63 72.77,6.93 71.27,6.93 U13_PIGGY.4 70.99,6.99 70.94,6.93 67.44,6.93 65.91,8.46 65.91,9.53 67.59,11.2 67.59,14.25 68.2,14.86 68.2,21.11 67.89,21.41 v67.89,28.42 | U13.10 25.25,48.84 22.94,48.84 22.48,48.39 v22.48,45.64 | v60.43,35.43 65.61,35.43 v66.06,35.89
N$118  (via drill 0.2)
  Top 0.152: v11.35,34.82 12.12,35.59 12.12,36.5 12.88,37.26 17.14,37.26 18.21,38.33 21.87,38.33 22.48,38.94 22.48,40.62 v22.94,41.07
  Bottom 0.152: RS8.R1B 10.36,33.76 11.05,33.76 11.35,34.06 v11.35,34.82 | U13.2 19.2,45.03 22.63,45.03 22.94,44.73 v22.94,41.07
N$119
  Bottom 0.152: RS11.R2A 10.37,50.52 12.12,50.52 12.57,50.06 17.14,50.06 17.45,49.76 17.45,47.93 17.75,47.62 U13.4
N$120
  Bottom 0.152: RS11.R1A 10.4,51.44 11.66,51.44 12.73,50.37 17.3,50.37 17.6,50.06 19.25,50.06 | 19.25,50.06 19.28,50.06 | 19.25,50.06 U13.6
N$121  (via drill 0.2)
  Top 0.152: v11.35,36.2 12.73,37.57 16.99,37.57 18.06,38.63 21.72,38.63 22.17,39.09 22.17,41.22 22.63,41.68 v24.46,41.68
  Bottom 0.152: RS8.R4B 10.4,36.2 v11.35,36.2 | v24.46,41.68 23.55,42.6 23.55,46.1 23.85,46.41 25.25,46.41 U13.12
N$122  (via drill 0.2)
